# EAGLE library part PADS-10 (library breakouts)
PIN HEADER
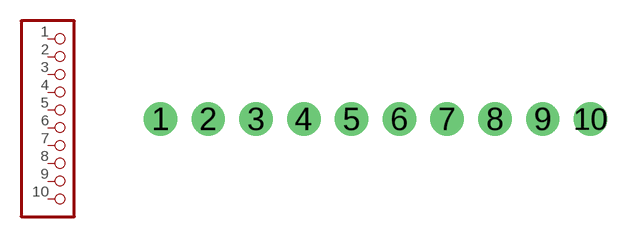
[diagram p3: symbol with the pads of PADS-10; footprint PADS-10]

Designator prefix JP

## PADS-10  [PADS-10]
1  1  pas
2  2  pas
3  3  pas
4  4  pas
5  5  pas
6  6  pas
7  7  pas
8  8  pas
9  9  pas
10  10  pas

## Footprint PADS-10 (pad centres in mm)
drill 1.016 pad 1.778: 1 -11.43,0; 2 -8.89,0; 3 -6.35,0; 4 -3.81,0; 5 -1.27,0; 6 1.27,0; 7 3.81,0; 8 6.35,0; 9 8.89,0; 10 11.43,0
